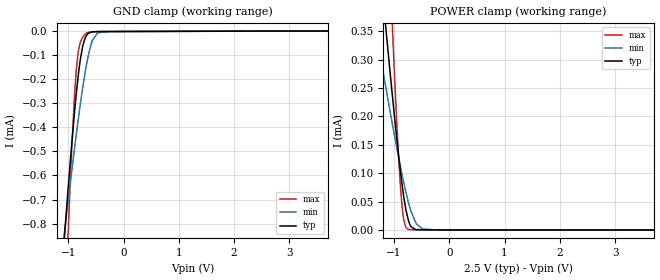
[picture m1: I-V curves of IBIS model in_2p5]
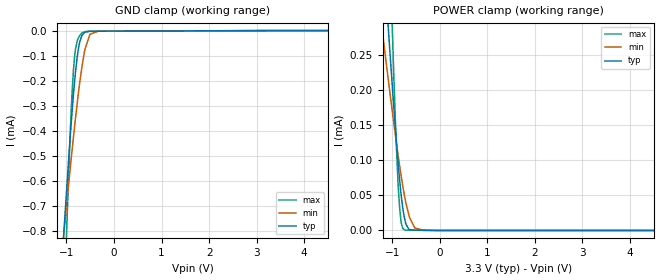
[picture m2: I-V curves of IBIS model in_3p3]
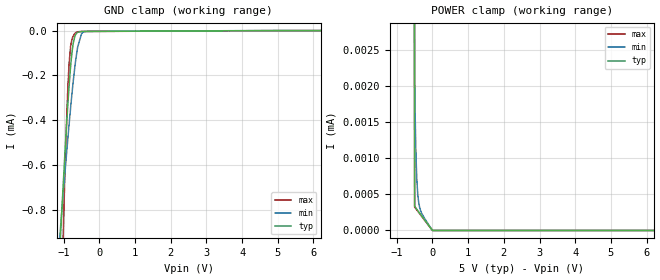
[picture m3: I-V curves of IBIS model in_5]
|Texas Instruments Incorporated
| High-Performance, 5.7kVRMS Reinforced Quad Channel Digital Isolators.
[IBIS Ver]   4.1
[File name]   iso7760.ibs
[File Rev]   2.0
[Date]   3/20/2018
[Source]
| Texas Instruments Incorporated.
| Analog-eLab Design Center, HPA
| 12500 TI Blvd
| Dallas, TX -75243
[Notes]   Revision History:
| Rev 2.0: 3/20/2018
| _ Clean up the header
| Rev 1.0: 7/20/2017
| - Initial version of the model
| - Model based on ISO7840
| - C_comp although listed in numerical order of value are
|   obtained from varying PVT conditions. For PVT conditions for
|   each specific value refer the buffer description under
|   respective [Model]. IBIS model user is responsible for using
|   appropriate C_comp to simulate for Signal Integrity.
|* EXCEPTION:   *
|* - For in_* and en_* models there will be leakage current in   *
|*   GROUND clamp because of a resistor(RH2) connected to pad.   *
|* - For inf_* models there will be leakage current in POWER clamp  *
|*   because of a resistor(R1) connected to pad.   *
[Disclaimer]
| This model is designed as an aid for customers of Texas Instruments.
| TI and its licensors and suppliers make no warranties, either expressed
| or implied, with respect to this  model, including the warranties of
| merchantability or fitness for a particular purpose. The model is
| provided solely on an "as is" basis. The entire risk as to its quality
| and performance is with the customer.
[Copyright]
(C) Copyright 2016 Texas Instruments Incorporated.All rights reserved.
|   IS07760DW
[Component]   IS07760DW
[Manufacturer]   TI
[Package]   |16 SOIC - DW package
|   typ   min   max
R_pkg   0.13983   0.12494   0.17928
L_pkg   2.1802nH   1.92454nH   2.85707nH
C_pkg   0.42060pF   0.21450pF   0.61276pF
[Pin]  signal_name   model_name   R_pin   L_pin   C_pin
1   VCC1   POWER   0.09703   2.25823nH  0.63889pF
2   INA   IN   0.10567   2.15194nH  0.30706pF
3   INB   IN   0.12889   1.99554nH  0.21450pF
4   INC   IN   0.12623   1.94755nH  0.61276pF
5   IND   IN   0.12494   1.92646nH  0.36666pF
6   INE   IN   0.14038   2.18765nH  0.43235pF
7   INF   IN   0.17807   2.83638nH  0.45904pF
8   GND1   GND   0.08216   2.43955nH  0.44498pF
9   GND2   GND   0.10126   2.44074nH  0.40934pF
10   OUTF   OUT   0.17928   2.85707nH  0.52717pF
11   OUTE   OUT   0.12883   1.99615nH  0.50841pF
12   OUTD   OUT   0.12617   1.94399nH  0.32633pF
13   OUTC   OUT   0.12498   1.92454nH  0.37783pF
14   OUTB   OUT   0.14050   2.18615nH  0.38097pF
15   OUTA   OUT   0.08275   2.09014nH  0.75096pF
16   VCC2   POWER   0.09747   2.26909nH  0.67439pF
|   IS07760FDW
[Component]   IS07760FDW
[Manufacturer]   TI
[Package]   |16 SOIC - DW package
|   typ   min   max
R_pkg   0.13983   0.12494   0.17928
L_pkg   2.1802nH   1.92454nH   2.85707nH
C_pkg   0.42060pF   0.21450pF   0.61276pF
[Pin]  signal_name   model_name   R_pin   L_pin   C_pin
1   VCC1   POWER   0.09703   2.25823nH  0.63889pF
2   INA   INF   0.10567   2.15194nH  0.30706pF
3   INB   INF   0.12889   1.99554nH  0.21450pF
4   INC   INF   0.12623   1.94755nH  0.61276pF
5   IND   INF   0.12494   1.92646nH  0.36666pF
6   INE   INF   0.14038   2.18765nH  0.43235pF
7   INF   INF   0.17807   2.83638nH  0.45904pF
8   GND1   GND   0.08216   2.43955nH  0.44498pF
9   GND2   GND   0.10126   2.44074nH  0.40934pF
10   OUTF   OUT   0.17928   2.85707nH  0.52717pF
11   OUTE   OUT   0.12883   1.99615nH  0.50841pF
12   OUTD   OUT   0.12617   1.94399nH  0.32633pF
13   OUTC   OUT   0.12498   1.92454nH  0.37783pF
14   OUTB   OUT   0.14050   2.18615nH  0.38097pF
15   OUTA   OUT   0.08275   2.09014nH  0.75096pF
16   VCC2   POWER   0.09747   2.26909nH  0.67439pF
|   IS07760DBQ
[Component]   IS07760DBQ
[Manufacturer]   TI
[Package]   |16 SSOP - DBQ package
|   typ   min   max
R_pkg   0.063   0.035   0.092
L_pkg   1.606n   1.484n   1.943n
C_pkg   0.292p   0.236p   0.522p
[Pin]  signal_name   model_name   R_pin   L_pin   C_pin
1   VCC1   POWER   0.03488  1.48406n  0.34063p
2   INA   IN   0.09199  1.94262n  0.52214p
3   INB   IN   0.07362  1.68527n  0.25393p
4   INC   IN   0.06934  1.61924n  0.25014p
5   IND   IN   0.06434  1.54435n  0.24552p
6   INE   IN   0.06312  1.52800n  0.24436p
7   INF   IN   0.06469  1.55584n  0.24569p
8   GND1   GND   0.04061  1.49221n  0.23623p
9   GND2   GND   0.04264  1.49221n  0.48652p
10   OUTF   OUT   0.06469  1.55584n  0.24589p
11   OUTE   OUT   0.06312  1.52800n  0.24463p
12   OUTD   OUT   0.06434  1.54435n  0.24576p
13   OUTC   OUT   0.06934  1.61924n  0.25041p
14   OUTB   OUT   0.07362  1.68527n  0.25423p
15   OUTA   OUT   0.08996  1.94262n  0.27232p
16   VCC2   POWER   0.03488  1.48406n  0.34107p
|   IS07760FDBQ
[Component]   IS07760FDBQ
[Manufacturer]   TI
[Package]   |16 SSOP - DBQ package
|   typ   min   max
R_pkg   0.063   0.035   0.092
L_pkg   1.606n   1.484n   1.943n
C_pkg   0.292p   0.236p   0.522p
[Pin]  signal_name   model_name   R_pin   L_pin   C_pin
1   VCC1   POWER   0.03488  1.48406n  0.34063p
2   INA   INF   0.09199  1.94262n  0.52214p
3   INB   INF   0.07362  1.68527n  0.25393p
4   INC   INF   0.06934  1.61924n  0.25014p
5   IND   INF   0.06434  1.54435n  0.24552p
6   INE   INF   0.06312  1.52800n  0.24436p
7   INF   INF   0.06469  1.55584n  0.24569p
8   GND1   GND   0.04061  1.49221n  0.23623p
9   GND2   GND   0.04264  1.49221n  0.48652p
10   OUTF   OUT   0.06469  1.55584n  0.24589p
11   OUTE   OUT   0.06312  1.52800n  0.24463p
12   OUTD   OUT   0.06434  1.54435n  0.24576p
13   OUTC   OUT   0.06934  1.61924n  0.25041p
14   OUTB   OUT   0.07362  1.68527n  0.25423p
15   OUTA   OUT   0.08996  1.94262n  0.27232p
16   VCC2   POWER   0.03488  1.48406n  0.34107p
|   Model Selectors
[Model Selector] IN
in_2p5   2.5V digital Input
in_3p3   3.3V digital Input
in_5   5.0V digital Input
[Model Selector] INF
inf_2p5   2.5V digital Input
inf_3p3   3.3V digital Input
inf_5   5.0V digital Input
[Model Selector] OUT
out_2p5   2.5V digital 3-state
out_3p3   3.3V digital 3-state
out_5   5.0V digital 3-state
| Models and submodels in the file (9): in_2p5 (Input), in_3p3 (Input), in_5 (Input), inf_2p5 (Input), inf_3p3 (Input), inf_5 (Input), out_2p5 (3-state), out_3p3 (3-state), out_5 (3-state)
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|   in_2p5 Model
[Model]   in_2p5
Model_type   Input
Vinl = 0.75
Vinh = 1.75
|   typ   min   max
|   (nom PVT)   (fast PVT)   (slow PVT)
C_comp   3.281e-15   3.281e-15   3.250e-14
[Model spec]
|subparameter
Vinl   0.75   0.675   0.825
Vinh   1.75   1.575   1.925
| Where nom  PVT is Nominal Process, 2.5V, 27C
|   Fast PVT is Strong Process,  2.75V, -55C
|   Slow PVT is Weak Process,   2.25V, 150C
[Voltage Range]   2.5   2.25   2.75
|Ambient Temperature   25   125   -55
|Junction Temperature
[Temperature Range]   27   150   -55
[Power Clamp Reference]   2.5   2.25   2.75
[GND Clamp Reference]   0   0   0
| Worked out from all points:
|   GND clamp passes 1 mA (typ) near -1.12 V on its own axis
[GND Clamp]
|   Voltage   I(typ)   I(min)   I(max)
-2.5V     -5.567mA   -3.855mA   -11.2mA
-1.071V   -859.9uA   -843.3uA   -1.249mA
-1.015V   -691.9uA   -732.5uA   -914.2uA
-965mV    -547.7uA   -635.6uA   -635.6uA
-894mV    -356.2uA   -501.7uA   -297uA
-827.5mV  -201.6uA   -381.9uA   -101.5uA
-737.5mV  -61.36uA   -233.7uA   -24.74uA
-643.8mV  -10.62uA   -108.8uA   -5.86uA
-564mV    -3.337uA   -39.15uA   -2.62uA
-468.2mV  -2.078uA   -7.417uA   -2.095uA
-250mV    -1.826uA   -1.892uA   -1.932uA
5V        0A         0A         0A
[POWER Clamp]
|   Voltage   I(typ)   I(min)   I(max)
-2.5V     1.812mA    1.039mA    3.985mA
-1.351V   565.2uA    364.2uA    1.113mA
-1.196V   404.1uA    277.3uA    740.6uA
-1.053V   258.8uA    198.6uA    407.1uA
-990.2mV  197.6uA    165uA      269.2uA
-924.3mV  136.7uA    131uA      139.5uA
-874.8mV  94.88uA    106.6uA    63.72uA
-822.5mV  56.84uA    82.23uA    17.11uA
-740mV    16.82uA    48.51uA    910.2nA
-612.5mV  771.4nA    14.03uA    395.2nA
-486.3mV  326.4nA    1.63uA     313.2nA
5V        0A         0A         0A
|   in_3p3 Model
[Model]   in_3p3
Model_type   Input
Vinl = 0.99
Vinh = 2.31
|   typ   min   max
|   (nom PVT)   (fast PVT)   (slow PVT)
C_comp   3.281e-15   3.281e-15   3.329e-14
[Model spec]
|subparameter
Vinl   0.99   0.891   1.089
Vinh   2.31   2.079   2.541
| Where nom  PVT is Nominal Process, 3.3V, 27C
|   Fast PVT is Strong Process,  3.63V, -55C
|   Slow PVT is Weak Process,   2.97V, 150C
[Voltage Range]   3.3   2.97   3.63
|Ambient Temperature   25   125   -55
|Junction Temperature
[Temperature Range]   27   150   -55
[Power Clamp Reference]   3.3   2.97   3.63
[GND Clamp Reference]   0   0   0
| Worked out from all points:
|   GND clamp passes 1 mA (typ) near -1.12 V on its own axis
|   POWER clamp passes 1 mA (typ) near -1.76 V on its own axis
[GND Clamp]
|   Voltage   I(typ)   I(min)   I(max)
-3.3V     -8.284mA   -5.57mA    -16.97mA
-1.076V   -873.8uA   -852.4uA   -1.277mA
-1.002V   -654.6uA   -707.6uA   -841.1uA
-893.3mV  -354.6uA   -500.5uA   -294.5uA
-853.4mV  -258.1uA   -427.8uA   -159.9uA
-825mV    -196.7uA   -377.6uA   -97.46uA
-772.2mV  -104.4uA   -288.5uA   -41.12uA
-722.7mV  -47.98uA   -211.7uA   -20.38uA
-620.4mV  -7.55uA    -84.56uA   -4.818uA
-505.2mV  -2.819uA   -14.66uA   -2.744uA
-330mV    -2.413uA   -2.673uA   -2.551uA
6.6V      0A         0A         0A
[POWER Clamp]
|   Voltage   I(typ)   I(min)   I(max)
-3.3V     2.693mA    1.517mA    6.009mA
-1.242V   451.1uA    302.7uA    849uA
-1.198V   405.5uA    278.1uA    743.9uA
-1.049V   255uA      196.5uA    398.4uA
-965.9mV  174.7uA    152.3uA    218.9uA
-878.8mV  98.13uA    108.5uA    68.84uA
-842.5mV  70.44uA    91.34uA    30.66uA
-805.2mV  46.22uA    74.6uA     9.403uA
-737.2mV  15.94uA    47.51uA    852.4nA
-526mV    364.9nA    3.505uA    338.9nA
-330mV    219.3nA    268.9nA    212.6nA
6.6V      0A         0A         0A
|   in_5 Model
[Model]   in_5
Model_type   Input
Vinl = 1.5
Vinh = 3.5
|   typ   min   max
|   (nom PVT)   (fast PVT)   (slow PVT)
C_comp   3.281e-15   3.281e-15   3.455e-14
[Model spec]
|subparameter
Vinl   1.5   1.35   1.65
Vinh   3.5   3.15   3.85
| Where nom  PVT is Nominal Process, 5V, 27C
|   Fast PVT is Strong Process,  5.5V, -55C
|   Slow PVT is Weak Process,   4.5V, 150C
[Voltage Range]   5   4.5   5.5
|Ambient Temperature   25   125   -55
|Junction Temperature
[Temperature Range]   27   150   -55
[Power Clamp Reference]   5   4.5   5.5
[GND Clamp Reference]   0   0   0
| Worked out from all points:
|   GND clamp passes 1 mA (typ) near -1.12 V on its own axis
[GND Clamp]
|   Voltage   I(typ)   I(min)   I(max)
-5V       -13.99mA   -9.044mA   -29.25mA
-1.112V   -984.6uA   -924.8uA   -1.503mA
-1.062V   -832.2uA   -825.1uA   -1.194mA
-974mV    -573.5uA   -653.1uA   -684.8uA
-908mV    -392.7uA   -527.9uA   -356.7uA
-850mV    -250.8uA   -421.9uA   -151.8uA
-809mV    -166.1uA   -350.2uA   -74.38uA
-740mV    -65.1uA    -237.9uA   -26.95uA
-608mV    -7.374uA   -73.42uA   -5.426uA
-500mV    -3.903uA   -14.37uA   -3.931uA
-338mV    -3.55uA    -3.864uA   -3.762uA
10V       0A         0A         0A
[POWER Clamp]
|   Voltage   I(typ)   I(min)   I(max)
-5V       185.5mA    66.86mA    305.6mA
-1.007V   213.6uA    173.9uA    305uA
-500mV    338.3nA    2.124uA    322.2nA
-482mV    323.5nA    1.505uA    310.6nA
-473mV    316.7nA    1.273uA    304.8nA
-459.5mV  306.8nA    1.002uA    296.1nA
-432.5mV  288nA      655.7nA    278.7nA
-396.5mV  263.7nA    427.3nA    255.5nA
-360.5mV  239.7nA    320.4nA    232.3nA
-306.5mV  203.8nA    241.2nA    197.5nA
-500uV    0A         0A         0A
10V       0A         0A         0A
